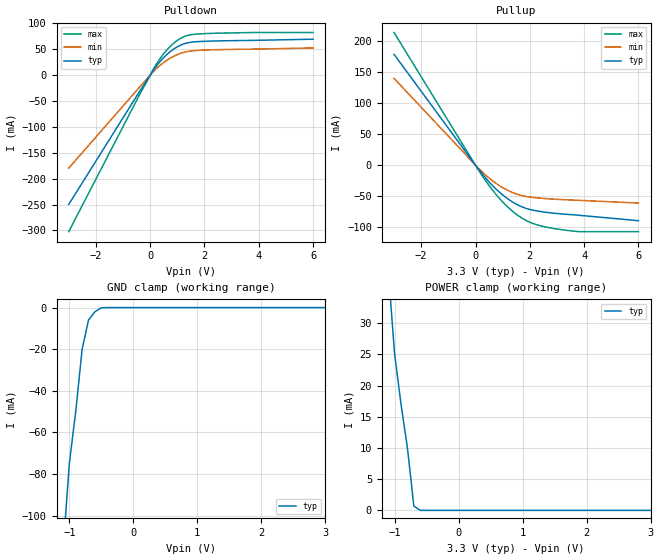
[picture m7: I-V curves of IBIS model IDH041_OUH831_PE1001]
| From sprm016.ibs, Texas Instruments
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[Model]   IDH041_OUH831_PE1001
Model_type   I/O
Polarity   Non-Inverting
Enable   Active-Low
| signals   A, GZ, Y
Vinl = 0.8V
Vinh = 2.0V
Cref = 30p
Rref = 50
Vref = 1.5
Vmeas = 1.5
|   typ   min   max
C_comp   6.2461p   6.1086p   6.8040p
|   typ   min   max
[Temperature Range]   25.0   0   90
|   typ   min   max
[Voltage Range]   3.3V   3.13V   3.47V
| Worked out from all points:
|   slope of the pulldown table from 0 to 0.495 V, typ, clamps not added: 14.6 ohm
|   slope of the pullup table from 0 to 0.495 V, typ, clamps not added: 18.6 ohm
|   GND clamp passes 1 mA (typ) near -0.55 V on its own axis
|   POWER clamp passes 1 mA (typ) near -0.70 V on its own axis
[Pulldown]
|   Voltage   I(typ)   I(min)   I(max)
-3V       -249.9mA   -179.7mA   -302.4mA
-400mV    -32.23mA   -23.71mA   -38.54mA
100mV     8.094mA    5.782mA    9.853mA
300mV     22.32mA    16.02mA    27.18mA
500mV     34.15mA    24.59mA    41.63mA
700mV     43.81mA    31.65mA    53.51mA
900mV     51.52mA    37.29mA    63.08mA
1.1V      57.42mA    41.63mA    70.51mA
1.3V      61.45mA    44.74mA    75.6mA
1.8V      64.87mA    47.98mA    79.65mA
3.8V      67.22mA    50.29mA    82.29mA
6V        69.42mA    52.49mA    82.3mA
[GND_clamp]
|   Voltage   I(typ)   I(min)   I(max)
-3V       -900mA     NA         NA
-2V       -500mA     NA         NA
-1V       -75mA      NA         NA
-900mV    -50mA      NA         NA
-800mV    -20mA      NA         NA
-700mV    -6mA       NA         NA
-600mV    -2mA       NA         NA
-500mV    -120uA     NA         NA
-400mV    0A         NA         NA
3V        0A         NA         NA
[Pullup]
|   Voltage   I(typ)   I(min)   I(max)
-3V       179mA      140.2mA    214.2mA
200mV     -11.43mA   -8.867mA   -13.79mA
500mV     -26.86mA   -20.62mA   -32.66mA
800mV     -40.16mA   -30.51mA   -49.29mA
1.1V      -51.31mA   -38.52mA   -63.59mA
1.4V      -60.23mA   -44.62mA   -75.51mA
1.8V      -68.6mA    -49.81mA   -87.57mA
2.1V      -72.31mA   -51.81mA   -93.67mA
2.5V      -75.34mA   -53.51mA   -98.76mA
3V        -77.84mA   -54.95mA   -102.9mA
3.8V      -80.65mA   -56.58mA   -107.1mA
6V        -89.45mA   -60.98mA   -107.1mA
[POWER_clamp]
|   Voltage   I(typ)   I(min)   I(max)
-3V       300mA      NA         NA
-2V       160mA      NA         NA
-1V       25mA       NA         NA
-900mV    17mA       NA         NA
-800mV    10mA       NA         NA
-700mV    700uA      NA         NA
-600mV    0A         NA         NA
-500mV    0A         NA         NA
3V        0A         NA         NA
[Ramp]
|   I(typ)   I(min)   I(max)
dV/dt_r   1.478/0.150n   1.234/0.200n   1.636/0.120n
dV/dt_f   1.400/0.170n   1.189/0.230n   1.557/0.140n
